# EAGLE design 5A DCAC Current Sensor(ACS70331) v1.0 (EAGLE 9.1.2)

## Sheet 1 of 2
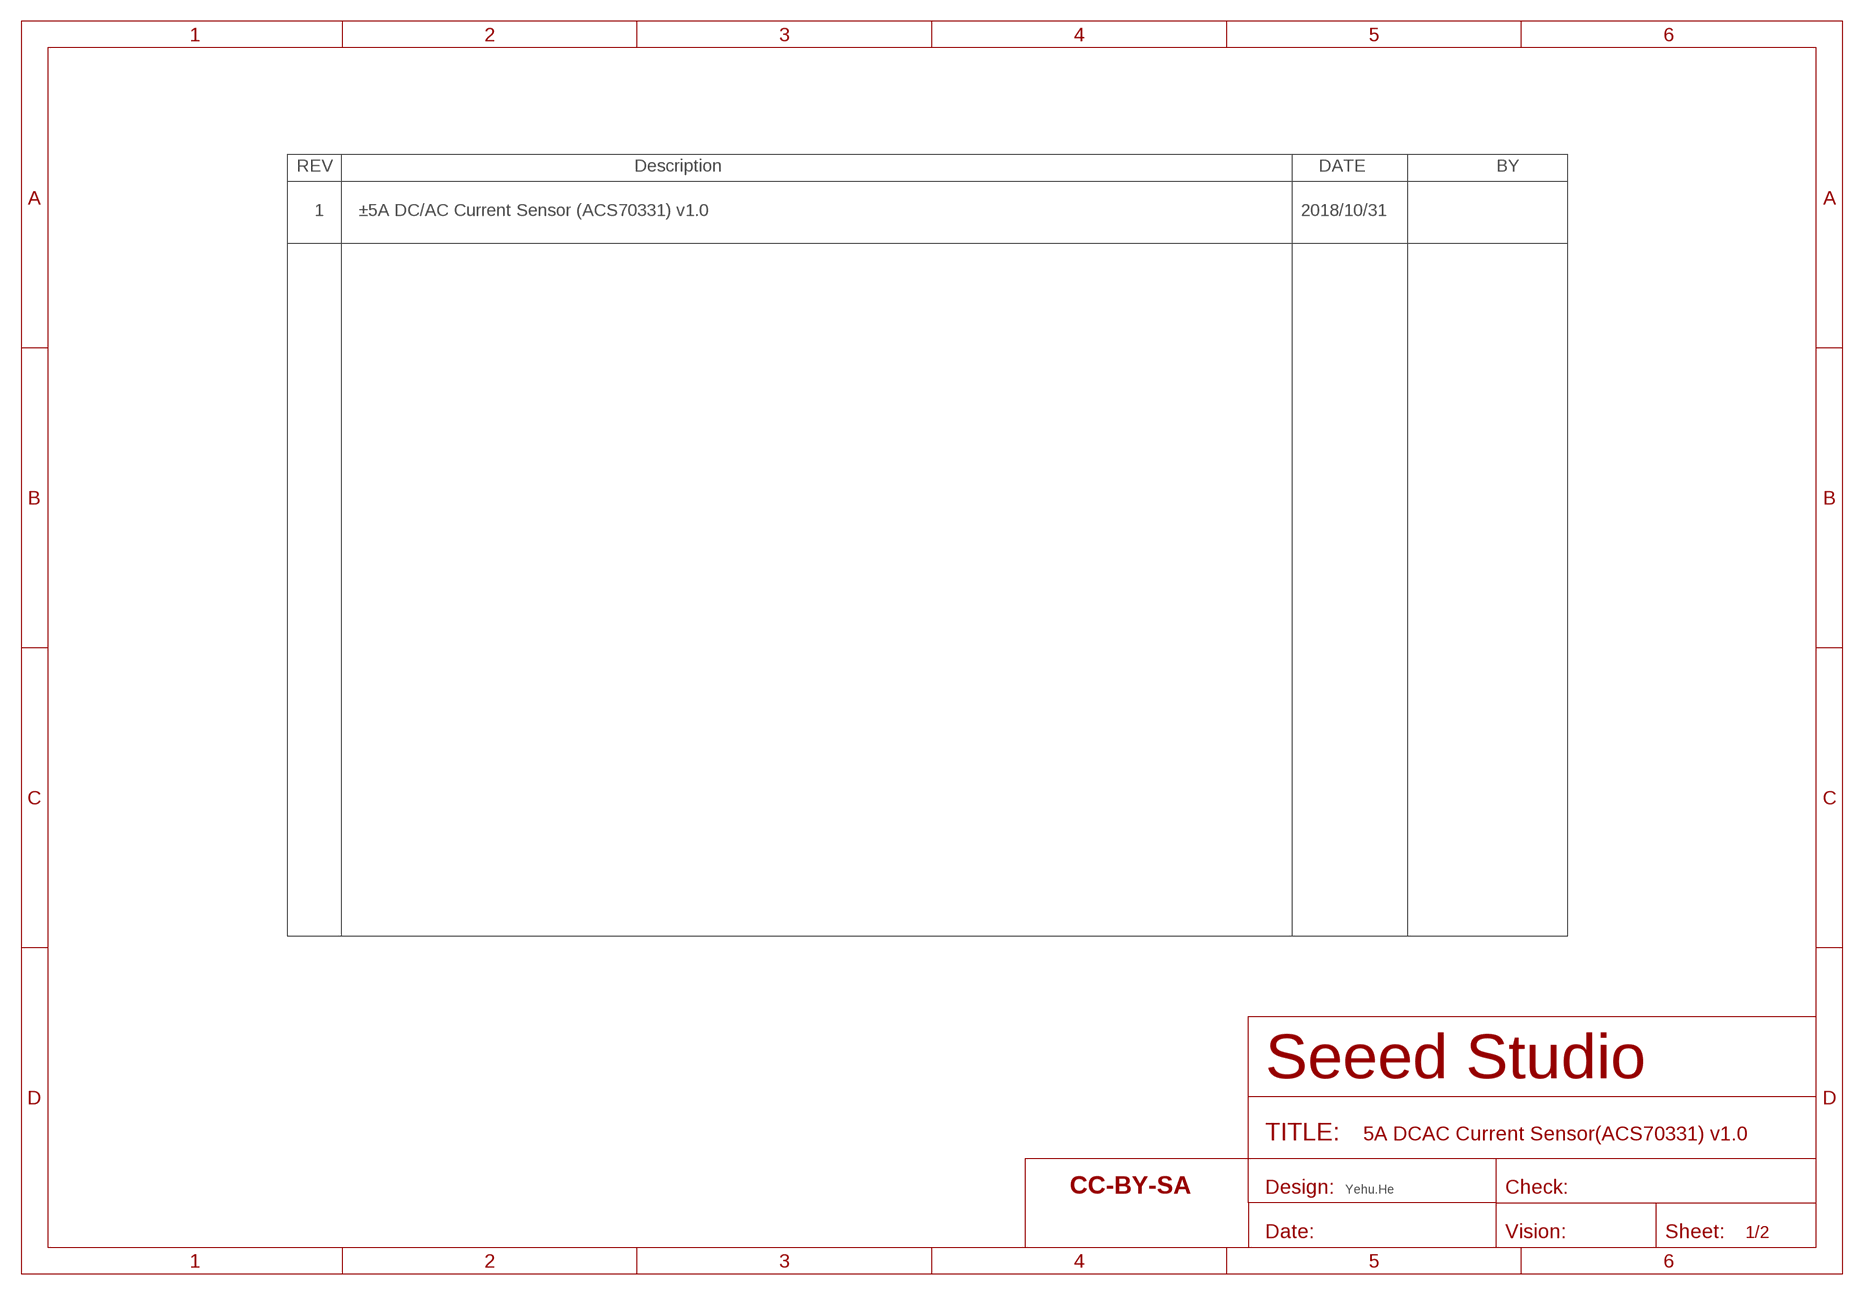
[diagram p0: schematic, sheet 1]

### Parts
FR1  SEEEDSTUDIO-OPEN-SCH-FRAME  [SEEEDSTUDIO-PCB-FRAME]

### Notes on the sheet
- 1 | ±5A DC/AC Current Sensor (ACS70331) v1.0 | 2018/10/31
- Yehu.He

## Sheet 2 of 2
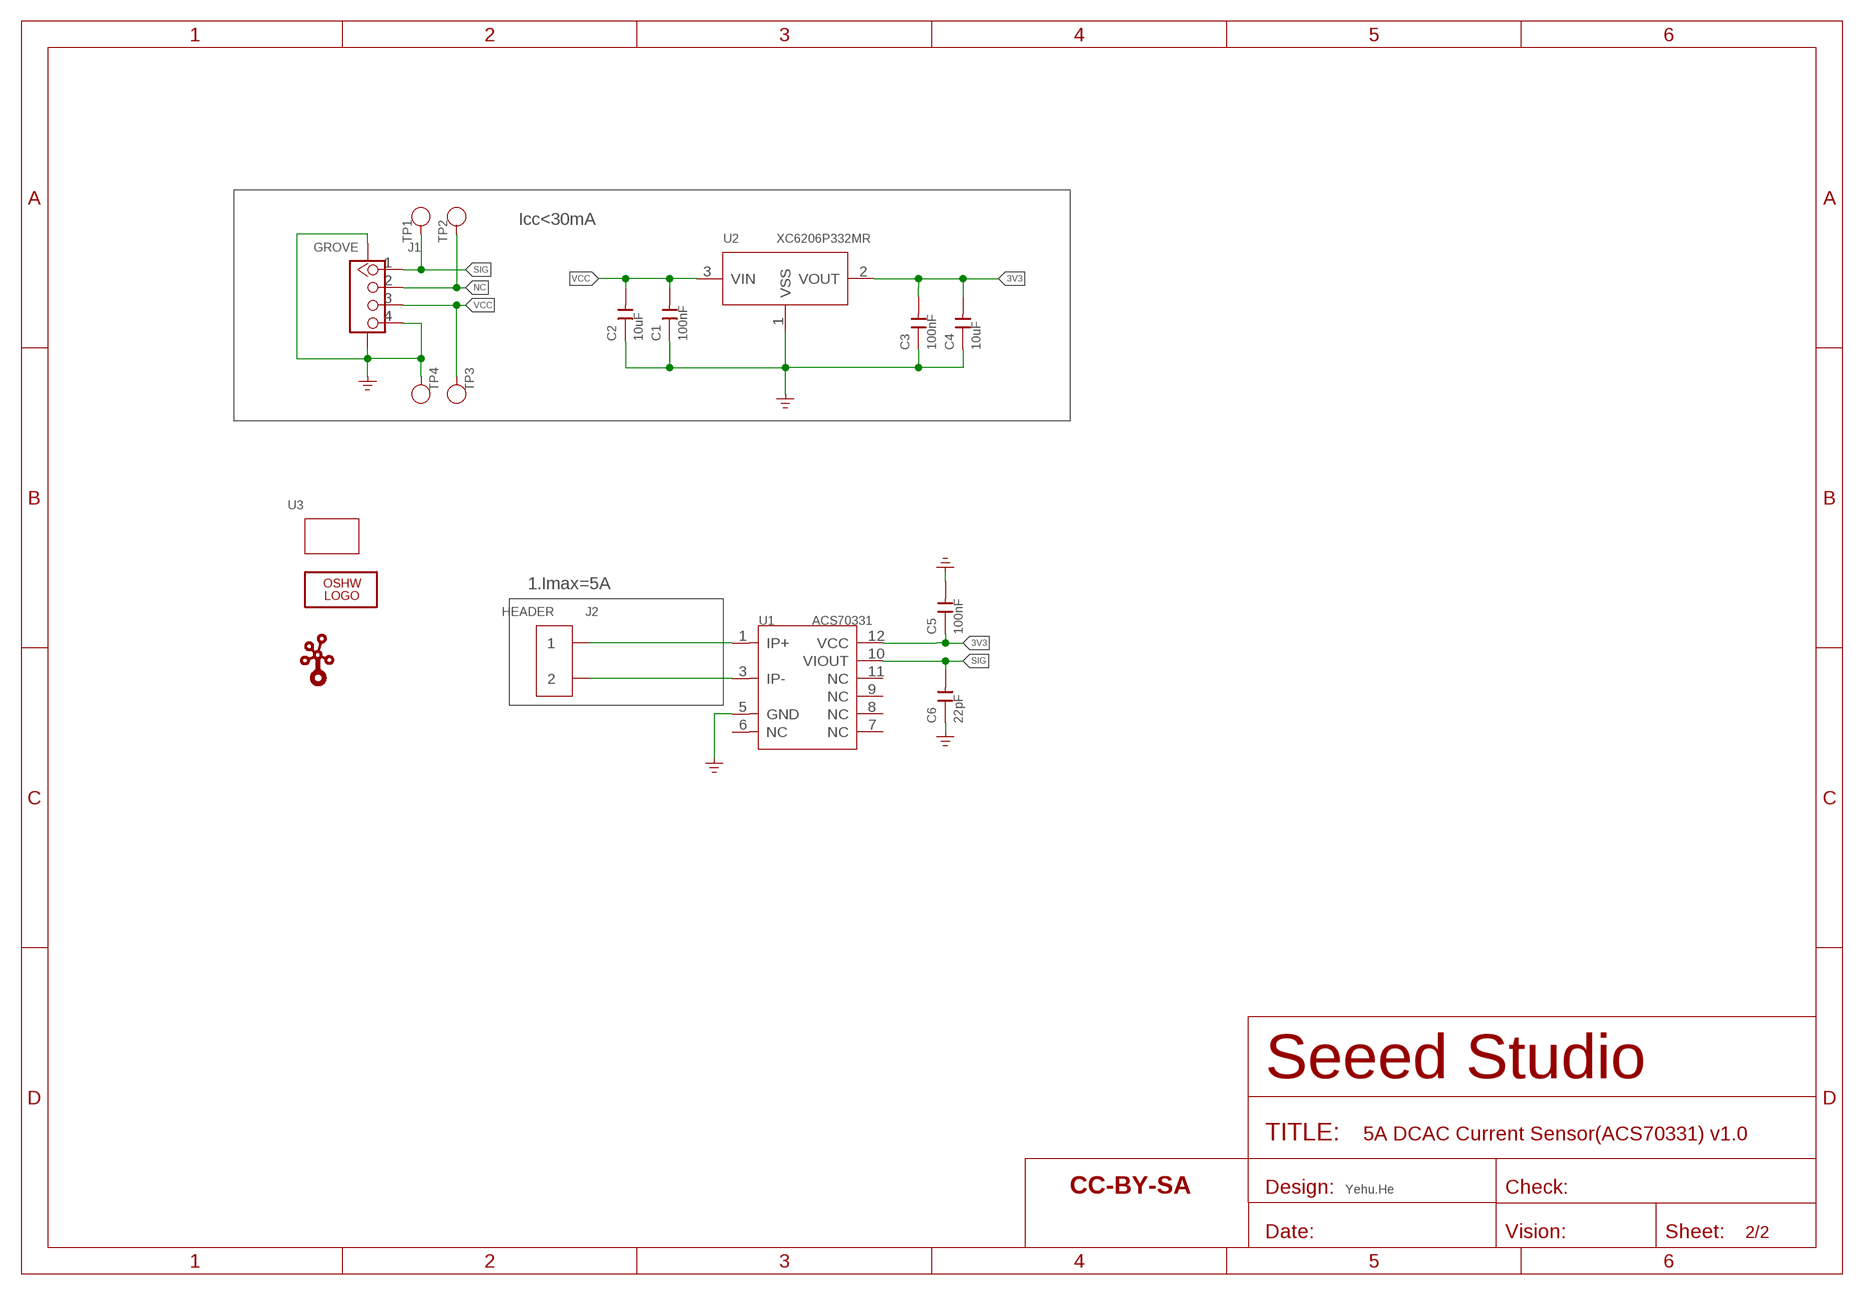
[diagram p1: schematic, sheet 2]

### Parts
C1  100nF  CAP-0603  [C0603]
C2  10uF  CAP-0603  [C0603]
C3  100nF  CAP-0603  [C0603]
C4  10uF  CAP-0603  [C0603]
C5  100nF  CAP-0603  [C0603]
C6  22pF  CAP-0603  [C0603]
FR2  SEEEDSTUDIO-OPEN-SCH-FRAME  [SEEEDSTUDIO-PCB-FRAME]
J1  GROVE  GROVE-CONNECTOR-SMD'DD'  [HW4-SMD-2.0]
J2  HEADER  SCREW-TERMINAL-2P'5.08'  [H2-5.0-10.5X8.0MM]
LOGO1  LOGO-OSHW-FILLX0200-NT  [OSHW_FILLX200_NOTEXT]
TP1  TEST-POINT'4545'  [TP-D45MIL]
TP2  TEST-POINT'4545'  [TP-D45MIL]
TP3  TEST-POINT'4545'  [TP-D45MIL]
TP4  TEST-POINT'4545'  [TP-D45MIL]
U1  ACS70331  SENSOR-ACS70331-QFN12  [QFN12-0.5-3X3X0.75MM]
U2  XC6206P332MR  PMIC-XC6206PMR  [SOT-23]
U3  GROVE-1X2-TOP  [GROVE-1*2-TEST-PLATFORM-TOP]
U$7  LOGO-GROVE  [GROVE-SILK-BIG]

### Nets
3V3: C3.2 C4.2 C5.1 U1.12(VCC) U2.2(VOUT)
GND: C1.1 C2.1 C3.1 C4.1 C5.2 C6.1 J1.4 J1.SS1 J1.SS2 TP4.T U1.5(GND) U2.1(VSS) ; supply symbol labelled GND_POWER
N$1: J2.1 U1.1(IP+)
N$2: J2.2 U1.3(IP-)
NC: J1.2 TP2.T
SIG: C6.2 J1.1 TP1.T U1.10(VIOUT)
VCC: C1.2 C2.2 J1.3 TP3.T U2.3(VIN)
Unconnected: U1.6(NC) U1.7(NC) U1.8(NC) U1.9(NC) U1.11(NC)

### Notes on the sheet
- Icc<30mA
- 1.Imax=5A
- Yehu.He

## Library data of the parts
C1-C6 = Discrete-new:CAP: Ceramic Capacitors
FR1 FR2 = moudle-new:SEEEDSTUDIO-OPEN-SCH-FRAME
J1 = Connector-new:GROVE-CONNECTOR-SMD: 4P-SMD-2.0:320110030;4P-SMD-2.0-90D:320110032
J2 = Connector-new:SCREW-TERMINAL-2P: 2P-3.5:320110028;2P-5.0:320110031
LOGO1 = logo:LOGO-OSHW-FILL; PARTNO: DNP
TP1-TP4 = Discrete-new:TEST-POINT; PARTNO: DNP
U1 = Discrete-new:SENSOR-ACS70331-QFN12
U2 = IC-new:PMIC-XC6206P: LOW ESR Cap.Compatible Positive Voltage Regulators
U3 = moudle-new:GROVE
U$7 = logo:LOGO-GROVE; PARTNO: DNP

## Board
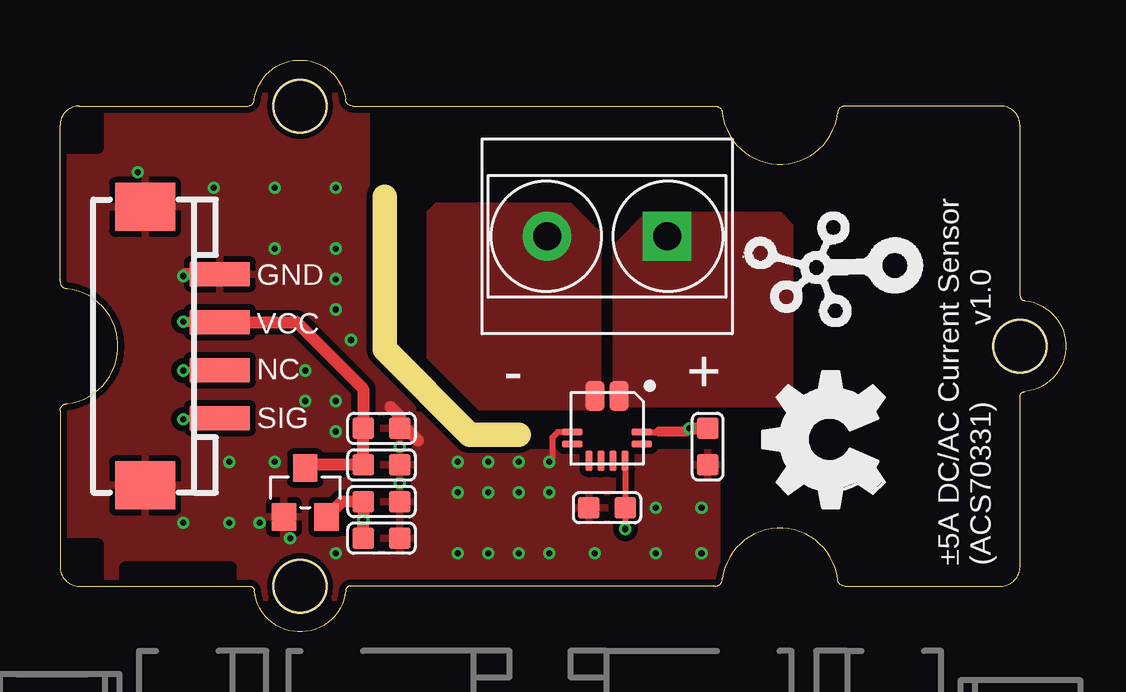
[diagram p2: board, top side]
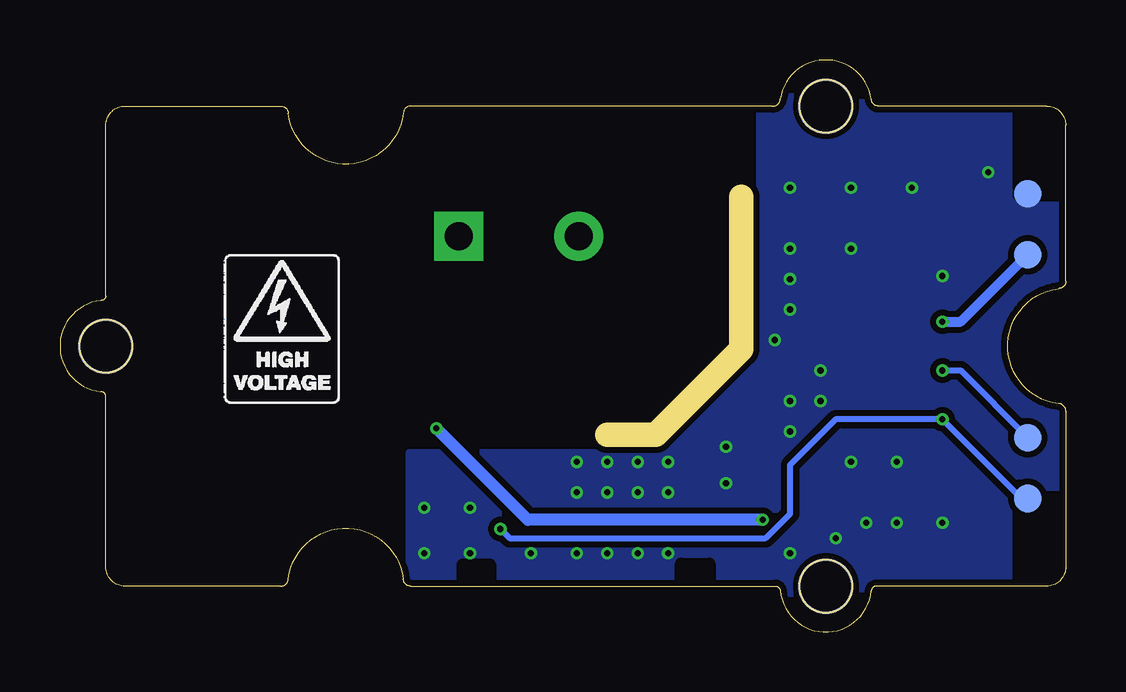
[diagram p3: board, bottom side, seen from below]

Size 41.91 x 23.83 mm. Coordinates in mm from the lower left corner, seen from the top.
Outline: 13.52,18.13 13.52,11.78 17.08,8.23 19.11,8.23
Copper layers (1*16): Top 0.035mm / dielectric 1.5mm / Bottom 0.035mm
Design rules "SeeedStudio_2layer_DRU_no_angle_20140221 *": minimum track width 1mil, minimum drill 10mil, track to track 6mil, track to pad 6mil, pad to pad 6mil, via to via 6mil, smd to smd 0mil, copper to edge 10mil, drill to drill 10mil, minimum pad ring 4mil, minimum via ring 4mil, stop-mask expansion 2mil, vias tented up to drill 25mil, thermal gap 10mil

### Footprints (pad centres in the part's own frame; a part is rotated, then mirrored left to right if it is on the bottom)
C0603 = smd 0.889 x 0.889: 1 0,0.762; 2 0,-0.762
HW4-SMD-2.0 = smd 1 x 2.5: 1 -3,0; 2 -1,0; 3 1,0; 4 3,0 | smd 2 x 2.5: SS1 -5.8,3.123; SS2 5.8,3.123
H2-5.0-10.5X8.0MM = drill 1.168 pad 2.032 square: 1 0,2.5 | drill 1.168 pad 2.032: 2 0,-2.5
TP-D45MIL = smd 1.143 x 1.143: T 0,0
QFN12-0.5-3X3X0.75MM = smd 1.27 x 0.8: 1 -1.35,0.5; 3 -1.35,-0.5 | smd 0.3 x 0.85: 5 0.15,-1.45; 6 0.65,-1.45; 11 0.65,1.45; 12 0.15,1.45 | smd 0.85 x 0.3: 7 1.35,-0.75; 8 1.35,-0.25; 9 1.35,0.25; 10 1.35,0.75
SOT-23 = smd 1.016 x 1.143: 1 -0.889,-1.016; 2 0.889,-1.016; 3 0,1.016
GROVE-1*2-TEST-PLATFORM-TOP = hole 2.2: 10.635,10; 10.635,-10; -19.365,0

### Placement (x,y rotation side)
C1  13.4,8.48 270 top
C2  13.4,6.96 270 top
C3  13.4,3.91 270 top
C4  13.4,5.43 270 top
C5  26.98,7.72 0 top
C6  22.79,5.18 90 top
FR1  not placed on the board
FR2  not placed on the board
J1  6.67,11.91 90 top
J2  22.79,16.48 270 top
LOGO1  34.35,5.18 90 top
TP1  1.58,5.56 0 bottom
TP2  1.58,8.1 0 bottom
TP3  1.58,15.72 0 bottom
TP4  1.58,18.26 0 bottom
U1  22.79,8.48 270 top
U2  10.22,5.81 0 top
U3  20.64,11.91 180 top
U$7  34.99,15.21 90 top

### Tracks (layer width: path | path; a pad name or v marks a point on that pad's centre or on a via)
3V3  (via drill 0.25 pad 0.51)
  Top 0.254: U1.12 24.93,8.33 24.95,8.35
  Top 0.406: 24.95,8.35 26.1,8.35 v26.22,8.48
  Top 0.508: v26.22,8.48 C5.1 | U2.2 11.74,5.43 C4.2 v12.63,4.67 C3.2
  Bottom 0.508: v26.22,8.48 22.41,4.67 v12.63,4.67
GND  (via drill 0.25 pad 0.51)
  Top 0.254: U1.5 20.74,8.33 20.51,8.1 20.51,7.21 v20.38,7.08
  Top 0.508: J1.4 5.22,14.91 v5.14,14.83 | 13.78,9.37 14.16,8.99 C1.1 14.41,8.48 14.92,7.97
  other vias: 3.24,19.15 6.41,18.51 11.49,18.51 8.95,18.51 11.49,15.97 8.95,15.97 5.14,4.54 7.05,4.54 7.05,7.08 8.32,4.54 8.95,7.08 11.49,14.7 11.49,13.43 12.13,12.16 14.16,7.72 14.16,6.19 16.57,7.08 17.84,7.08 19.11,7.08 19.11,5.81 17.84,5.81 16.57,5.81 20.38,3.27 20.38,5.81 19.11,3.27 17.84,3.27 16.57,3.27 11.49,3.27 9.59,3.91 22.29,3.27 24.83,3.27 26.73,3.27 26.73,5.18 24.83,5.18 10.22,10.89 10.22,9.62 11.49,8.35 11.49,9.62
  pour Bottom (isolate 0.254, rank 6): -0.57,22.32 12.76,22.32 12.76,11.4 16.7,7.46 27.37,7.46 27.37,1.37 -0.57,1.37
  pour Top (isolate 0.254, rank 6): -0.57,22.32 12.76,22.32 12.76,11.4 16.7,7.46 27.37,7.46 27.37,1.37 -0.57,1.37
N$1
  pour Top (isolate 0.254, no thermals): 23.05,9.37 23.05,16.1 24.45,17.5 30,17.5 30.54,16.96 30.54,9.91 30,9.37
N$2
  pour Top (isolate 0.254, no thermals): 22.29,9.24 17.46,9.24 15.3,11.4 15.3,17.5 15.68,17.88 21.27,17.88 22.54,16.61 22.54,9.5
NC  (via drill 0.25 pad 0.51)
  Top 0.254: J1.2 5.16,10.91 v5.14,10.89
  Bottom 0.254: v5.14,10.89 4.38,10.89 TP2.T
SIG  (via drill 0.25 pad 0.51)
  Top 0.254: U1.10 23.54,5.19 C6.2 v23.56,4.29 | J1.1 5.19,8.91 v5.14,8.86
  Bottom 0.254: TP1.T 1.84,5.56 v5.14,8.86 9.59,8.86 11.49,6.96 11.49,4.92 12.51,3.91 23.18,3.91 v23.56,4.29
VCC  (via drill 0.25 pad 0.51)
  Top 0.406: J1.3 5.16,12.91 v5.14,12.92
  Top 0.508: J1.3 9.86,12.91 12.63,10.13 C1.2 C2.2 10.35,6.96 U2.3
  Bottom 0.406: v5.14,12.92 4.38,12.92 TP3.T

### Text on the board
tNames: GND | VCC | NC | - | + | SIG | ±5A DC/AC Current Sensor / (ACS70331) v1.0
